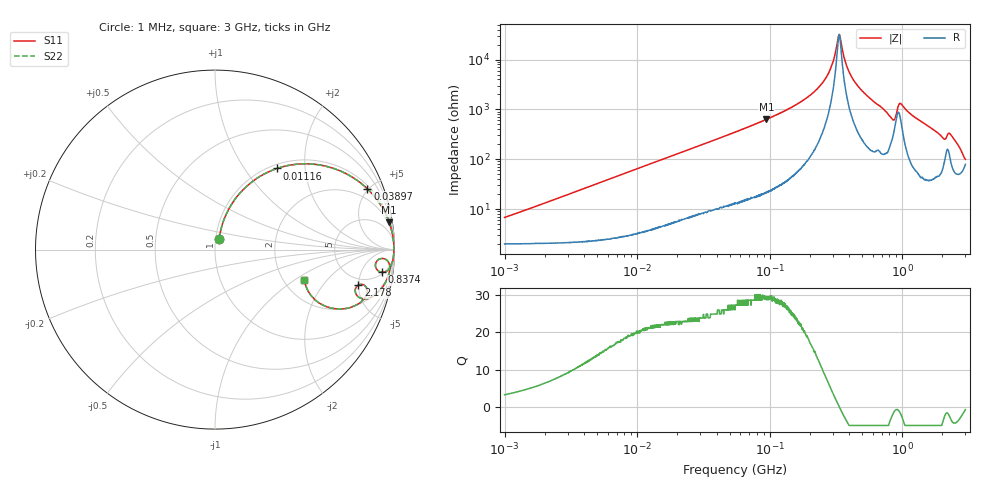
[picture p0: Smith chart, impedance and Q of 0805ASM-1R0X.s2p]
!s-Parameter Generated by FASTRON Sdn. Bhd.
!FASTRON P/N : 0805ASM-1R0X
!Keysight Technologies: E4991B_MY54100416_A.01.15
!Date: Fri Jun 19 14:53:56 2026
!Version  :Rev00  Fri Jun 19 14:53:56 2026
!Data & Calibration Information:
!Freq  S11  S21  S12  S22
!PortZ  Port1:50+j0  Port2:50+j0
!When reading reference impedance value at option line is always used.
! Remarks : This data is being provided solely for informational purposes.
# Hz S dB R 50
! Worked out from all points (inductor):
!   1601 points, 1 MHz to 3 GHz, reference 50 ohm
!   read as one part in series: L = 1.03 uH near 1.041 MHz
!   highest Q = 29.7 at 94.5 MHz (marker M1), where L = 1.06 uH
!   self-resonance near 333.5 MHz
!   S11 on the Smith chart (normalised r, x): 1 MHz: 1.04, +0.13; 11.16 MHz: 1.07, +1.43; 38.97 MHz: 1.20, +4.94; 837.4 MHz: 6, -12; 2.178 GHz: 4.06, -4.98; 3 GHz: 2.58, -1.21
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1000000  -23.60 69.2  -0.19 -3.6  -0.19 -3.6  -23.60 69.2
3804036  -12.60 71.4  -0.43 -13.5  -0.43 -13.5  -12.60 71.4
1.115534e7  -4.88 52.5  -2.00 -34.7  -2.00 -34.7  -4.88 52.5
1.447069e7  -3.54 45.7  -2.89 -41.6  -2.89 -41.6  -3.54 45.7
3.897472e7  -0.78 21.7  -8.63 -66.0  -8.63 -66.0  -0.78 21.7
5.504702e7  -0.42 15.8  -11.30 -72.1  -11.30 -72.1  -0.42 15.8
9.450168e7  -0.15 9.0  -16.10 -79.1  -16.10 -79.1  -0.15 9.0
2.083556e8  -0.04 2.8  -26.30 -83.7  -26.30 -83.7  -0.04 2.8
2.785165e8  -0.03 1.1  -34.60 -79.8  -34.60 -79.8  -0.03 1.1
3.351655e8  -0.03 -0.0  -50.10 0.4  -50.10 0.4  -0.03 -0.0
3.817355e8  -0.03 -0.8  -37.40 74.8  -37.40 74.8  -0.03 -0.8
4.347762e8  -0.04 -1.5  -31.40 80.5  -31.40 80.5  -0.04 -1.5
7.925923e8  -0.29 -7.1  -18.00 71.2  -18.00 71.2  -0.29 -7.1
8.374426e8  -0.56 -7.7  -16.80 60.5  -16.80 60.5  -0.56 -7.7
8.71647e8  -0.89 -6.6  -16.70 45.1  -16.70 45.1  -0.89 -6.6
9.779672e8  -0.31 -3.8  -22.60 59.8  -22.60 59.8  -0.31 -3.8
1.511446e9  -0.30 -11.2  -14.20 74.3  -14.20 74.3  -0.30 -11.2
1.980367e9  -0.99 -17.8  -10.10 61.2  -10.10 61.2  -0.99 -17.8
2.177892e9  -1.69 -13.9  -11.00 44.5  -11.00 44.5  -1.69 -13.9
2.492946e9  -1.32 -20.3  -8.99 56.8  -8.99 56.8  -1.32 -20.3
2.769173e9  -2.70 -26.5  -6.46 43.6  -6.46 43.6  -2.70 -26.5
3e9  -5.58 -18.8  -5.52 18.7  -5.52 18.7  -5.58 -18.8
